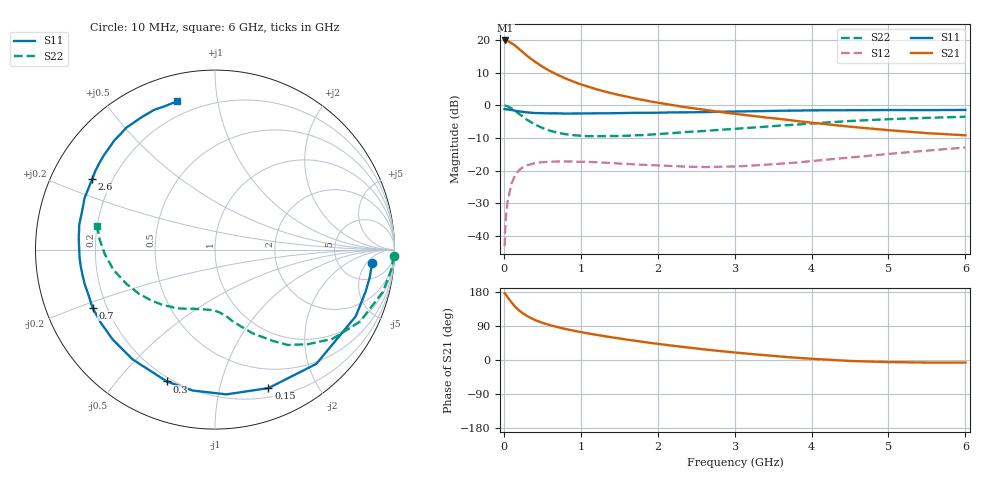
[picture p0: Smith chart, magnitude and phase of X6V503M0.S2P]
! SIEMENS Small Signal Semiconductors
! BFP193W
! Si NPN RF Bipolar Junction Transistor in SOT343
! VCE = 0.5 V  IC = 3 mA
! Common Emitter S-Parameters:  April 1994
# GHz  S  MA  R  50
!  f  S11  S21  S12  S22
! GHz  MAG  ANG  MAG  ANG  MAG  ANG  MAG  ANG
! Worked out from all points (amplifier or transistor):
!   40 points, 10 MHz to 6 GHz, reference 50 ohm
!   highest |S21| = 19.9 dB at 20 MHz (marker M1)
!   |S21| within 3 dB of that: start of sweep to 217.2 MHz
!   unconditionally stable (mu >= 1): 1.79 GHz to end of sweep
!   at 200 MHz: K = 0.12, MSG = 18.6 dB, |S12| = -19.9 dB
!   at 1.5 GHz: K = 0.85, MSG = 10.5 dB, |S12| = -17.9 dB
!   at 6 GHz: K = 1.18, MAG = -0.7 dB, |S12| = -12.9 dB
!   S11 on the Smith chart (normalised r, x): 10 MHz: 11, -7; 150 MHz: 0.29, -1.42; 300 MHz: 0.18, -0.68; 700 MHz: 0.15, -0.22; 2.6 GHz: 0.13, +0.26; 6 GHz: 0.13, +0.77
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0.01  0.8787 -5.0  9.88 176.3  0.0069 87.7  0.9955 -2.0
0.02  0.8758 -10.2  9.935 174.1  0.0141 83.7  0.9903 -5.9
0.05  0.8678 -25.3  9.717 165.4  0.0342 76.6  0.965 -14.1
0.1  0.8511 -48.4  9.054 152.0  0.0634 63.8  0.9022 -26.4
0.15  0.8271 -68.9  8.224 140.0  0.0858 53.5  0.822 -37.2
0.2  0.8091 -85.5  7.313 130.5  0.1016 45.3  0.739 -45.5
0.25  0.7951 -99.1  6.529 122.8  0.1129 38.6  0.6688 -52.6
0.3  0.7821 -110.1  5.8 116.2  0.1203 33.5  0.6042 -57.5
0.4  0.7647 -127.0  4.726 106.0  0.1295 25.7  0.5123 -65.7
0.5  0.7586 -138.8  3.942 98.2  0.1344 20.5  0.4513 -71.4
0.6  0.7557 -147.6  3.364 91.9  0.1366 16.4  0.4091 -76.4
0.7  0.7549 -154.7  2.947 86.7  0.1376 13.8  0.3801 -79.8
0.9  0.7511 -165.4  2.331 77.7  0.1374 9.7  0.3491 -86.3
1.1  0.7538 -173.0  1.936 70.0  0.1354 6.9  0.3366 -92.0
1.3  0.7564 -179.7  1.648 63.2  0.132 5.1  0.3367 -97.5
1.6  0.7645 172.1  1.363 53.7  0.1266 4.5  0.3422 -104.7
2.2  0.7814 158.5  1.007 37.6  0.1169 7.4  0.3758 -119.1
2.6  0.7885 150.2  0.858 28.1  0.1134 12.0  0.4039 -128.4
3.2  0.8127 139.3  0.698 16.1  0.1186 20.3  0.4536 -141.3
4.5  0.8433 119.2  0.471 -2.5  0.1585 30.4  0.5763 -168.6
5.5  0.8464 109.2  0.375 -6.7  0.2022 29.8  0.6446 175.1
6  0.8525 104.5  0.348 -6.9  0.2258 28.1  0.6695 168.7
